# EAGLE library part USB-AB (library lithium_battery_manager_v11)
This is a USB AB connector that is compatible with USB OTG. i.e. this connector can serve as a host or device
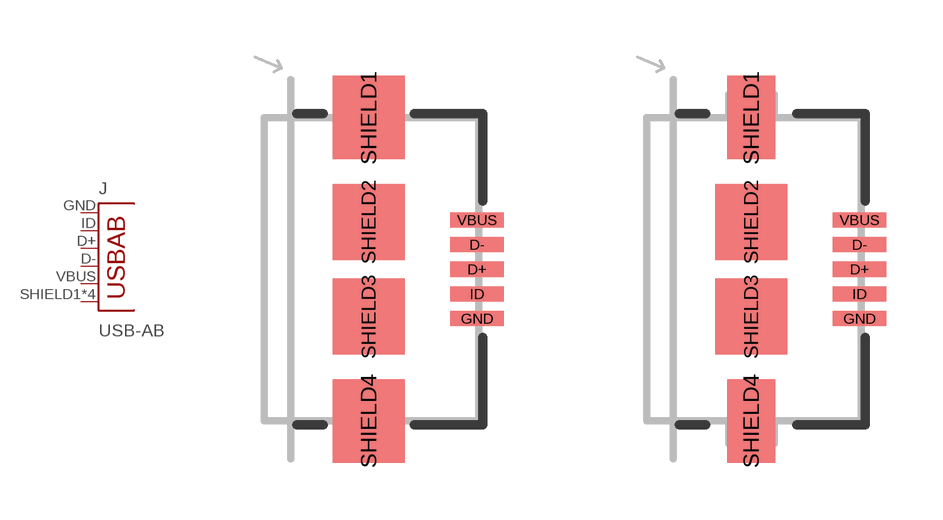
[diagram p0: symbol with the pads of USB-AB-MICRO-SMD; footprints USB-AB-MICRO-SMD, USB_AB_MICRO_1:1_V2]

Designator prefix J

## USB-AB  [USB-AB-MICRO-SMD]
D+  D+
D-  D-
GND  GND
ID  USBID
SHIELD1  SHIELD
SHIELD2  SHIELD
SHIELD3  SHIELD
SHIELD4  SHIELD
VBUS  VBUS

## USB-AB"  [USB_AB_MICRO_1:1_V2]
Pads as for USB-AB-MICRO-SMD

## USB-ABCONN-11794 (PROD_ID: CONN-11794)  [USB-AB-MICRO-SMD_V03]
D+1  D+
D-1  D-
GND1  GND
ID1  USBID
SHIELD1  SHIELD
SHIELD2  SHIELD
SHIELD3  SHIELD
VBUS1  VBUS

## Footprint USB-AB-MICRO-SMD (pad centres in mm)
micro USB AB connector for OTG support. 5-pins: USBVCC, GND, D+, D-, USBID. Can act as host or device
smd 1.4 x 0.4: D+ 2.85,0; D- 2.85,0.65; GND 2.85,-1.3; ID 2.85,-0.65; VBUS 2.85,1.3
smd 1.9 x 2.2: SHIELD1 0,4; SHIELD4 0,-4
smd 1.9 x 2: SHIELD2 0,1.25; SHIELD3 0,-1.25

## Footprint USB_AB_MICRO_1:1_V2 (pad centres in mm)
smd 1.4 x 0.4: D+ 2.85,0; D- 2.85,0.65; GND 2.85,-1.3; ID 2.85,-0.65; VBUS 2.85,1.3
smd 1.27 x 2.2: SHIELD1 0,4; SHIELD4 0,-4
smd 1.9 x 2: SHIELD2 0,1.25; SHIELD3 0,-1.25

## Footprint USB-AB-MICRO-SMD_V03 (pad centres in mm)
smd 1.4 x 0.4: D+1 2.7,0; D-1 2.7,0.65; GND1 2.7,-1.3; ID1 2.7,-0.65; VBUS1 2.7,1.3
smd 1.5 x 1.8: SHIELD1 0,3.68; SHIELD3 0,-3.68
smd 1.5 x 2.5: SHIELD2 0,0
hole 0.85 at 2.2,1.9
hole 0.85 at 2.2,-1.9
